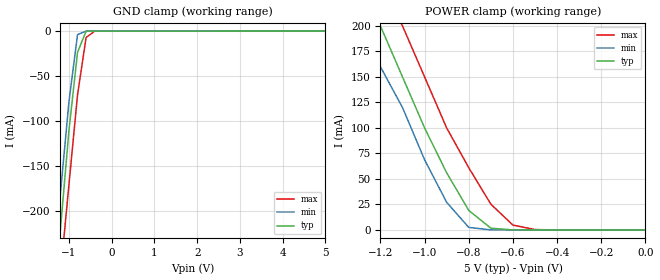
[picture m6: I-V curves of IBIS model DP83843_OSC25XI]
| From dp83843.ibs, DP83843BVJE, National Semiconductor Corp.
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|   Model OSC25XI
[Model]   DP83843_OSC25XI
Model_type   Input
Vinl =   0.80V
Vinh =   2.00V
Vmeas =   1.50V
C_comp   5.83pF   5.83pF   5.83pF
[Temperature Range]   50.00   -15.00   0.15k
[Voltage Range]   5.00V   4.50V   5.50V
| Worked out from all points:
|   GND clamp passes 1 mA (typ) near -0.61 V on its own axis
|   POWER clamp passes 1 mA (typ) near -0.65 V on its own axis
[GND_clamp]
| voltage   I(typ)   I(min)   I(max)
-5V       -2.37A     -2.34A     -2.42A
-1.4V     -330mA     -290mA     -380mA
-1.2V     -220mA     -180mA     -270mA
-1V       -110mA     -77.9mA    -170mA
-800mV    -23.44mA   -3.81mA    -70.7mA
-600mV    -170uA     -63.82uA   -7.09mA
-400mV    -47.22uA   -60.47uA   -91.52uA
5V        43.94uA    62.5uA     27.83uA
[POWER_clamp]
| voltage   I(typ)   I(min)   I(max)
-5V       2.16A      2.13A      2.2A
-1.3V     240mA      210mA      290mA
-1.2V     200mA      160mA      240mA
-1.1V     150mA      120mA      200mA
-1V       100mA      68.79mA    150mA
-900mV    56mA       27.09mA    100mA
-800mV    19.14mA    2.53mA     61mA
-700mV    1.77mA     98.82uA    25.3mA
-600mV    100uA      64.12uA    4.78mA
-500mV    49.81uA    62.5uA     420uA
0V        43.94uA    56.25uA    30.61uA
